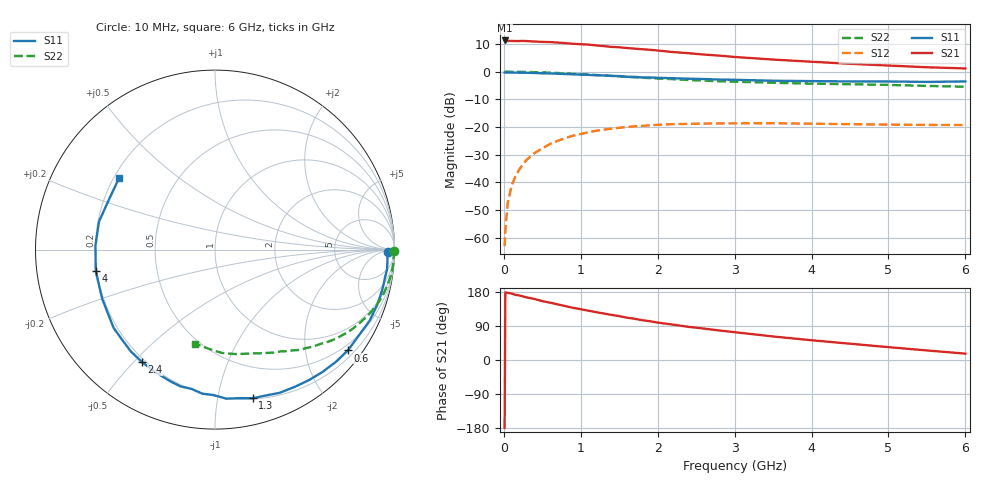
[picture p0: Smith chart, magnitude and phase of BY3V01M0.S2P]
! SIEMENS Small Signal Semiconductors
! BFY420
! Si NPN RF SIEGET Grounded Emitter Transistor in MICRO-X
! VCE = 3 V  IC = 1 mA
! Common Emitter S-Parameters:  October  1996
# GHz  S  MA  R  50
!  f  S11  S21  S12  S22
! GHz  MAG  ANG  MAG  ANG  MAG  ANG  MAG  ANG
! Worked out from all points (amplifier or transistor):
!   36 points, 10 MHz to 6 GHz, reference 50 ohm
!   highest |S21| = 11.3 dB at 10 MHz (marker M1)
!   |S21| within 3 dB of that: start of sweep to 1.718 GHz
!   unconditionally stable (mu >= 1): 4.513 GHz to end of sweep
!   at 250 MHz: K = 0.04, MSG = 22.3 dB, |S12| = -33.5 dB
!   at 1.4 GHz: K = 0.19, MSG = 14.8 dB, |S12| = -20.6 dB
!   at 6 GHz: K = 1.33, MAG = 6.8 dB, |S12| = -19.3 dB
!   S11 on the Smith chart (normalised r, x): 10 MHz: 48, -18; 600 MHz: 0.36, -2.93; 1.3 GHz: 0.21, -1.26; 2.4 GHz: 0.19, -0.53; 4 GHz: 0.20, -0.09; 6 GHz: 0.22, +0.32
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0.01  0.9643 -0.8  3.669 -179.4  0.0007 89.7  0.9985 -0.3
0.02  0.9602 -1.5  3.646 178.7  0.0014 80.7  0.9999 -0.5
0.05  0.9624 -3.1  3.582 177.0  0.0042 86.4  0.9987 -1.4
0.1  0.9649 -6.4  3.604 175.5  0.0086 86.7  0.9952 -2.9
0.15  0.9599 -9.4  3.574 171.9  0.0128 83.1  0.9954 -4.4
0.2  0.9589 -12.5  3.582 170.4  0.017 83.0  0.9947 -5.8
0.3  0.9549 -18.7  3.569 165.1  0.0258 78.8  0.9893 -8.8
0.4  0.9483 -24.7  3.51 161.0  0.0338 74.8  0.9809 -11.7
0.5  0.9332 -31.0  3.46 155.3  0.0411 71.5  0.9715 -14.5
0.6  0.9292 -37.2  3.427 151.3  0.0493 67.7  0.9599 -17.3
0.9  0.8958 -54.3  3.193 137.6  0.0696 57.4  0.9166 -24.9
1.1  0.8755 -65.7  3.086 130.1  0.0805 51.3  0.8856 -29.8
1.3  0.8541 -75.8  2.903 122.6  0.0896 45.3  0.8533 -34.0
1.8  0.7869 -99.6  2.544 105.0  0.1049 33.2  0.7781 -43.2
2.2  0.7602 -115.9  2.263 93.3  0.1124 25.1  0.7324 -49.7
2.4  0.7468 -123.1  2.159 87.6  0.1139 22.0  0.7064 -52.7
2.8  0.7205 -136.3  1.951 77.9  0.1162 16.1  0.6705 -57.9
3.5  0.6857 -156.4  1.656 62.1  0.1169 8.9  0.6308 -66.3
4  0.6753 -169.7  1.513 52.1  0.1147 5.3  0.6079 -72.5
4.5  0.6664 178.1  1.388 43.0  0.1124 2.7  0.5933 -78.9
5.5  0.6533 154.6  1.202 25.2  0.109 1.2  0.553 -93.8
6  0.6663 143.5  1.144 16.8  0.1086 2.1  0.5354 -102.2
